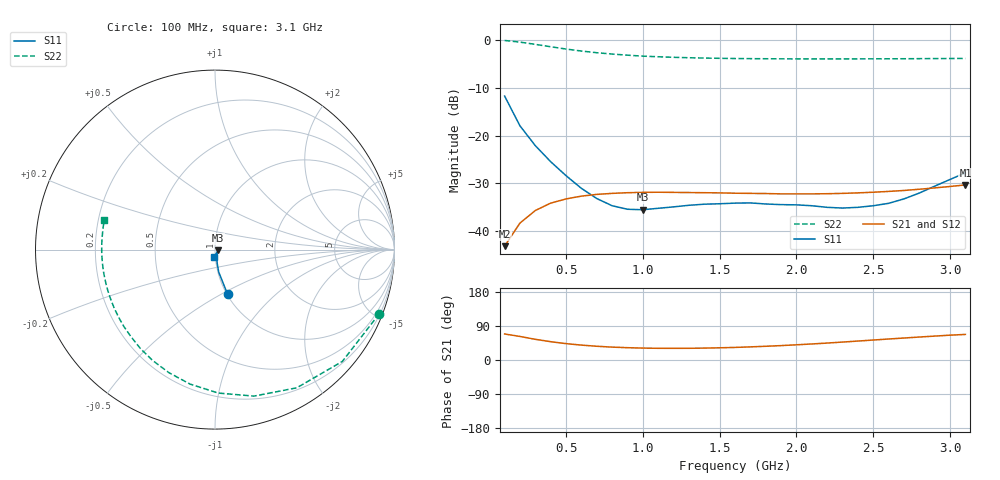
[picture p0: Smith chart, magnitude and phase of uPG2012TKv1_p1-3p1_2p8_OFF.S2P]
! NEC Compound Semiconductor Devices Ltd.
! 21.January 2005
! uPG2012TK
! GaAs MMIC (0.1 - 3.1GHz SPDT switch)
! VDD=2.8v Vcont=0v / IN-OUT1 ( OFF )
! OUT2:50ohm termination
#  GHz  S  MA  R  50
!  f  S11  S21  S12  S22
!  GHz  MAG  ANG  MAG  ANG  MAG  ANG  MAG  ANG
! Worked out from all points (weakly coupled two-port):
!   31 points, 100 MHz to 3.1 GHz, reference 50 ohm
!   highest |S21| = -30.31 dB at 3.1 GHz (marker M1); lowest = -43.1 dB at 100 MHz (marker M2)
!   lowest |S11| = -35.5 dB at 1 GHz (marker M3), VSWR 1.03, Z = 51.6 - j0.478 ohm
!   |S11| at or under -10 dB: start of sweep to end of sweep
!   |S22| runs from -4.0 to -0.2 dB; largest |S21 - S12| = 0.0004
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0.1  0.2582 -74.3  0.007 68.7  0.007 68.6  0.9828 -21.3
0.2  0.1262 -80.6  0.0122 62.1  0.0123 61.8  0.9442 -41.3
0.3  0.0784 -80.9  0.0165 54.6  0.0164 54.6  0.8947 -59.4
0.4  0.0533 -78.5  0.0197 48.3  0.0196 48.2  0.8447 -75.1
0.5  0.0381 -73.6  0.0218 43.2  0.0218 43.2  0.7995 -88.7
0.6  0.0281 -65.6  0.0233 39.3  0.0233 39.2  0.7621 -100.5
0.7  0.022 -54.4  0.0243 36.3  0.0242 36.2  0.732 -110.6
0.8  0.0185 -41.1  0.0249 34.0  0.0249 34.1  0.7087 -119.4
0.9  0.017 -27.4  0.0253 32.5  0.0252 32.6  0.69 -127.1
1  0.0168 -16.0  0.0255 31.4  0.0254 31.5  0.6741 -134.0
1.1  0.0174 -8.0  0.0256 30.9  0.0255 31.0  0.6642 -140.0
1.3  0.0187 0.3  0.0254 30.9  0.0254 31.1  0.6487 -150.2
1.6  0.0197 1.7  0.025 33.2  0.0251 33.3  0.6366 -162.3
1.7  0.0198 0.0  0.0249 34.6  0.0249 34.9  0.6347 -165.6
2.1  0.0185 -14.4  0.0246 42.3  0.0247 42.7  0.6311 -176.6
2.2  0.0178 -21.1  0.0247 44.7  0.0249 45.1  0.6313 -178.9
2.3  0.0175 -28.0  0.0249 47.3  0.0251 47.6  0.6313 178.9
2.4  0.0178 -37.0  0.0252 50.0  0.0253 49.5  0.6316 176.8
2.6  0.0196 -60.0  0.0261 55.4  0.0263 55.6  0.6326 173.1
2.7  0.0218 -70.3  0.0267 58.0  0.0269 58.3  0.6334 171.3
2.8  0.0251 -79.5  0.0275 60.6  0.0277 60.8  0.6346 169.6
3.1  0.0408 -101.1  0.0305 67.5  0.0309 67.5  0.6377 165.0
